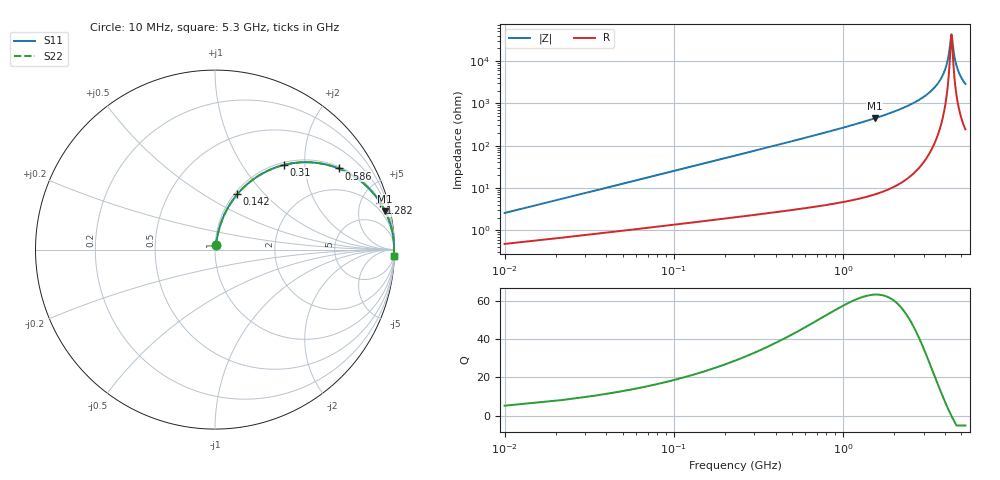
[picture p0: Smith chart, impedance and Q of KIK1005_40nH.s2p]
!version-3
!date-01.2023
!Series
# MHz S RI R 50
!Freq ReS11 ImS11 ReS21 ImS21 ReS12 ImS12 ReS22 ImS22
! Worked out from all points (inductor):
!   442 points, 10 MHz to 5.3 GHz, reference 50 ohm
!   read as one part in series: L = 40 nH near 34 MHz
!   highest Q = 63.2 at 1.546 GHz (marker M1), where L = 45.7 nH
!   self-resonance near 4.378 GHz
!   S11 on the Smith chart (normalised r, x): 10 MHz: 1.01, +0.05; 142 MHz: 1.03, +0.71; 310 MHz: 1.05, +1.57; 586 MHz: 1.07, +3.00; 1.282 GHz: 1.11, +7.05; 5.3 GHz: 6, -57
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10  0.00535 0.0249  0.9947 -0.0249  0.9947 -0.0249  0.00535 0.0249
46  0.0221 0.112  0.9779 -0.112  0.9779 -0.112  0.0221 0.112
70  0.0403 0.167  0.9597 -0.167  0.9597 -0.167  0.0403 0.167
142  0.124 0.308  0.876 -0.308  0.876 -0.308  0.124 0.308
310  0.3837 0.4715  0.6163 -0.4715  0.6163 -0.4715  0.3837 0.4715
586  0.6885 0.4523  0.3115 -0.4523  0.3115 -0.4523  0.6885 0.4523
898  0.8429 0.3549  0.1571 -0.3549  0.1571 -0.3549  0.8429 0.3549
1282  0.9219 0.2604  0.0781 -0.2604  0.0781 -0.2604  0.9219 0.2604
1546  0.9486 0.213  0.0514 -0.213  0.0514 -0.213  0.9486 0.213
1774  0.9633 0.1801  0.0367 -0.1801  0.0367 -0.1801  0.9633 0.1801
2662  0.9892 0.0931  0.0108 -0.0931  0.0108 -0.0931  0.9892 0.0931
3538  0.9964 0.039  0.00356 -0.039  0.00356 -0.039  0.9964 0.039
3814  0.9973 0.0252  0.00274 -0.0252  0.00274 -0.0252  0.9973 0.0252
4030  0.9976 0.0152  0.00241 -0.0152  0.00241 -0.0152  0.9976 0.0152
4210  0.9977 0.00729  0.00231 -0.00729  0.00231 -0.00729  0.9977 0.00729
4366  0.9977 0.000716  0.00233 -0.000716  0.00233 -0.000716  0.9977 0.000716
4390  0.9977 -0.000274  0.00234 0.000274  0.00234 0.000274  0.9977 -0.000274
4426  0.9976 -0.00175  0.00236 0.00175  0.00236 0.00175  0.9976 -0.00175
4546  0.9975 -0.00658  0.00247 0.00658  0.00247 0.00658  0.9975 -0.00658
4714  0.9973 -0.0131  0.0027 0.0131  0.0027 0.0131  0.9973 -0.0131
4966  0.9968 -0.0226  0.0032 0.0226  0.0032 0.0226  0.9968 -0.0226
5300  0.9959 -0.0344  0.00412 0.0344  0.00412 0.0344  0.9959 -0.0344
